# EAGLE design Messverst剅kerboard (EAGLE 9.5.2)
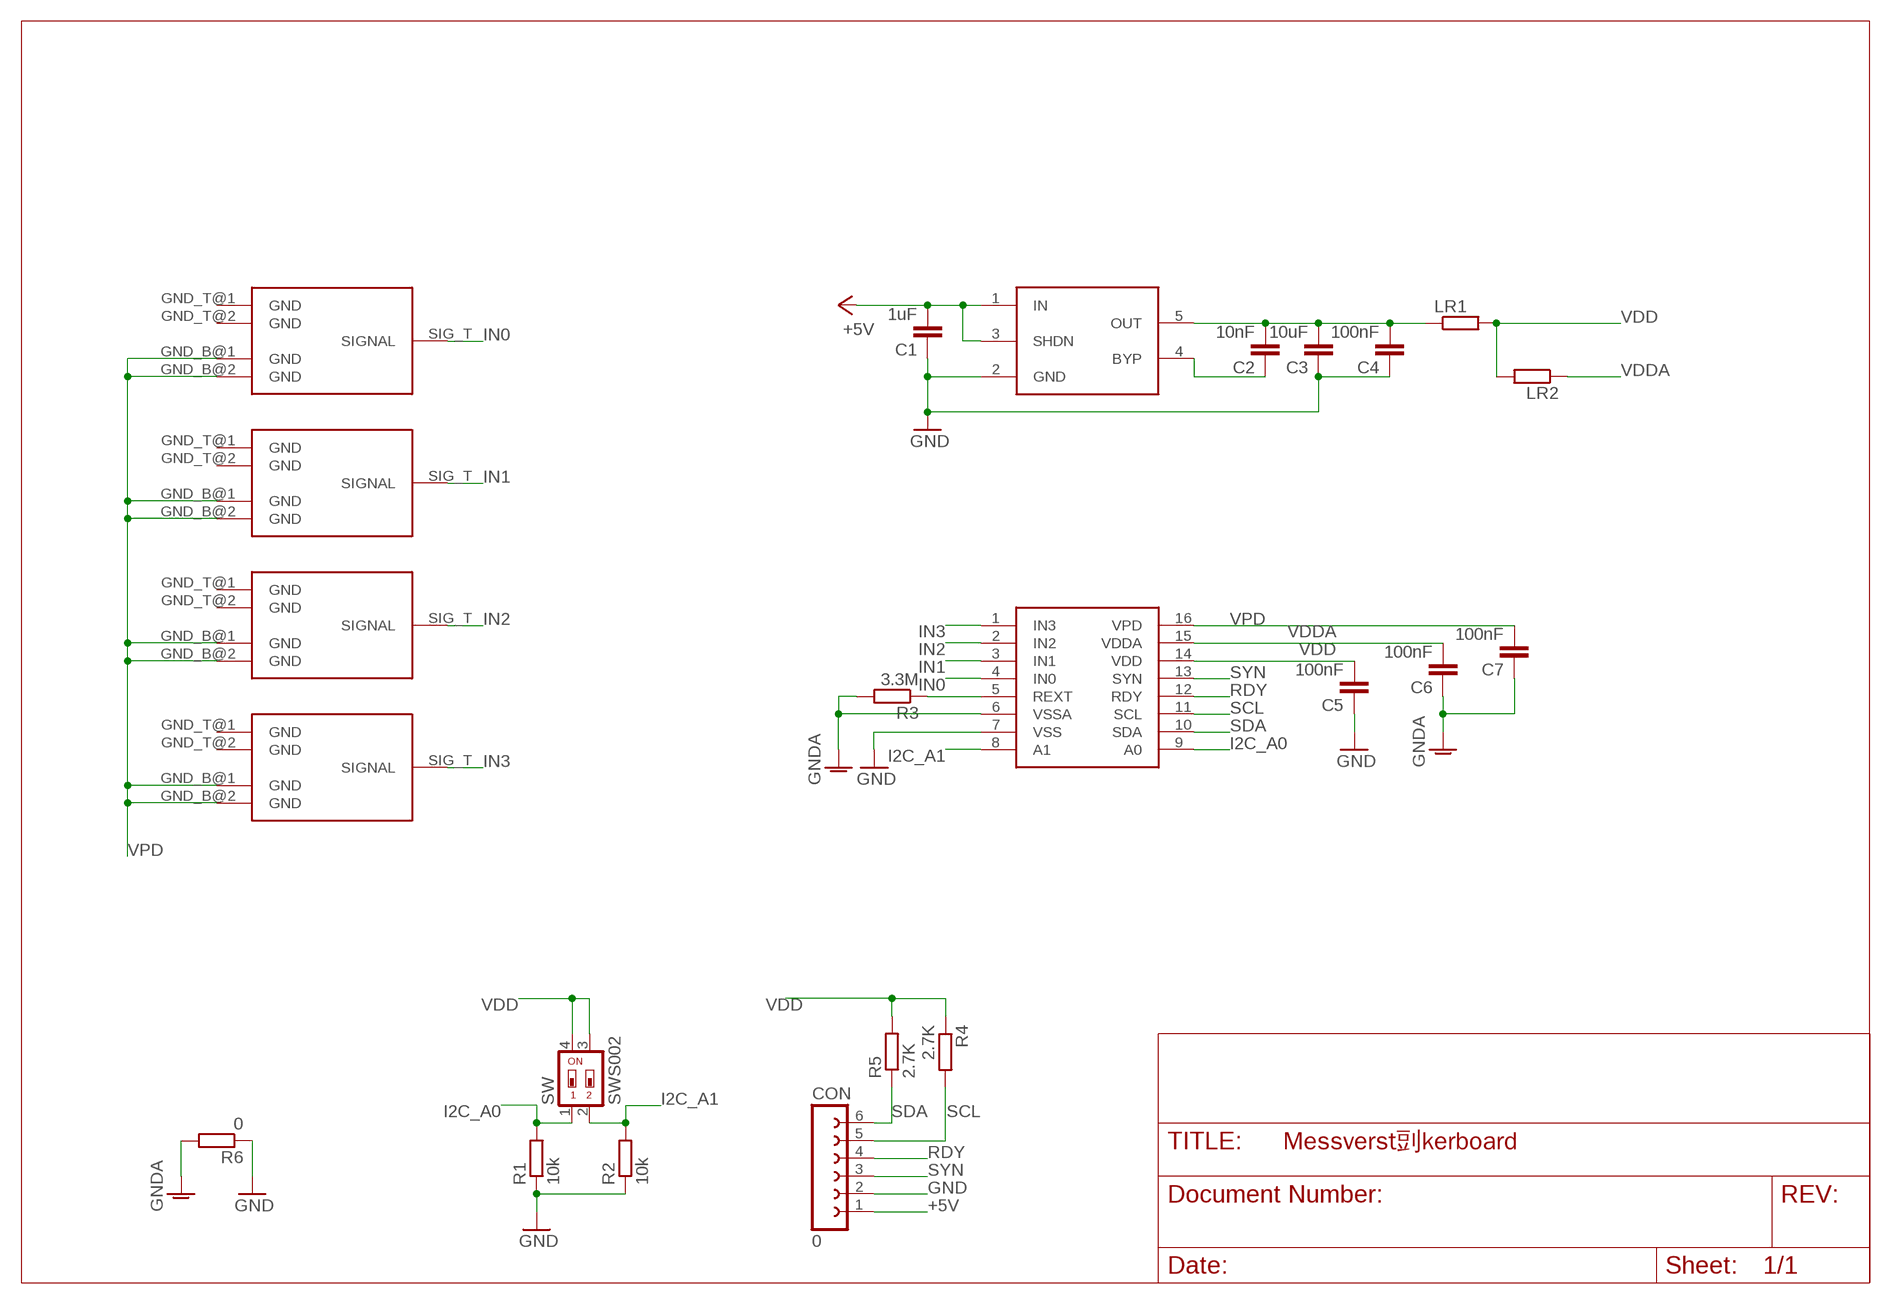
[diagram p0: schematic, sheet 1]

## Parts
AS89010  MCDC04  [SSOP16]
C1  1uF  C-EUC0603  [C0603]
C2  10nF  C-EUC0603  [C0603]
C3  10uF  C-EUC0603  [C0603]
C4  100nF  C-EUC0603  [C0603]
C5  100nF  C-EUC0603  [C0603]
C6  100nF  C-EUC0603  [C0603]
C7  100nF  C-EUC0603  [C0603]
CON  0  FE06-1  [FE06]
KANAL_1  SMA-BUCHSE-RANDMONTAGE  [SMA-RAND-PRINT]
KANAL_2  SMA-BUCHSE-RANDMONTAGE  [SMA-RAND-PRINT]
KANAL_3  SMA-BUCHSE-RANDMONTAGE  [SMA-RAND-PRINT]
KANAL_4  SMA-BUCHSE-RANDMONTAGE  [SMA-RAND-PRINT]
LDO  LT1761  [TSOT23-5]
LR1  R-EU_R0603  [R0603]
LR2  R-EU_R0603  [R0603]
R1  10k  R-EU_R0603  [R0603]
R2  10k  R-EU_R0603  [R0603]
R3  3.3M  R-EU_R0603  [R0603]
R4  2.7K  R-EU_R0603  [R0603]
R5  2.7K  R-EU_R0603  [R0603]
R6  0  R-EU_R0603  [R0603]
SW  SWS002  [SMS-002]

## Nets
+5V: C1.2 CON.1 LDO.1(IN) LDO.3(SHDN)
GND: AS89010.7(VSS) C1.1 C3.1 C4.1 C5.1 CON.2 LDO.2(GND) R1.1 R2.1 R6.1
GNDA: AS89010.6(VSSA) C6.1 C7.1 R3.2 R6.2
I2C_A0: AS89010.9(A0) R1.2 SW.1
I2C_A1: AS89010.8(A1) R2.2 SW.2
IN0: AS89010.4(IN0) KANAL_1.SIG_T(SIGNAL)
IN1: AS89010.3(IN1) KANAL_2.SIG_T(SIGNAL)
IN2: AS89010.2(IN2) KANAL_3.SIG_T(SIGNAL)
IN3: AS89010.1(IN3) KANAL_4.SIG_T(SIGNAL)
LDO_OUT3V3: C2.2 C3.2 C4.2 LDO.5(OUT) LR1.1
N$5: C2.1 LDO.4(BYP)
N$8: AS89010.5(REXT) R3.1
RDY: AS89010.12(RDY) CON.4
SCL: AS89010.11(SCL) CON.5 R4.2
SDA: AS89010.10(SDA) CON.6 R5.1
SYN: AS89010.13(SYN) CON.3
VDD: AS89010.14(VDD) C5.2 LR1.2 LR2.2 R4.1 R5.2 SW.3 SW.4
VDDA: AS89010.15(VDDA) C6.2 LR2.1
VPD: AS89010.16(VPD) C7.2 KANAL_1.GND_B@1(GND) KANAL_1.GND_B@2(GND) KANAL_2.GND_B@1(GND) KANAL_2.GND_B@2(GND) KANAL_3.GND_B@1(GND) KANAL_3.GND_B@2(GND) KANAL_4.GND_B@1(GND) KANAL_4.GND_B@2(GND)
Unconnected: KANAL_1.GND_T@1(GND) KANAL_1.GND_T@2(GND) KANAL_2.GND_T@1(GND) KANAL_2.GND_T@2(GND) KANAL_3.GND_T@1(GND) KANAL_3.GND_T@2(GND) KANAL_4.GND_T@1(GND) KANAL_4.GND_T@2(GND)

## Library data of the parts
AS89010 = BachelorLib:MCDC04
C1-C7 = rcl:C-EU: CAPACITOR, European symbol
CON = con-lsta:FE06-1: FEMALE HEADER; OC_FARNELL: unknown; OC_NEWARK: unknown
KANAL_1-KANAL_4 = OpenPhotonicsLib:SMA-BUCHSE-RANDMONTAGE
LDO = OpenPhotonicsLib:LT1761
LR1 LR2 R1-R6 = rcl:R-EU_: RESISTOR, European symbol
SW = smd-special:SWS002: SMD Dip Switch 2 pol.

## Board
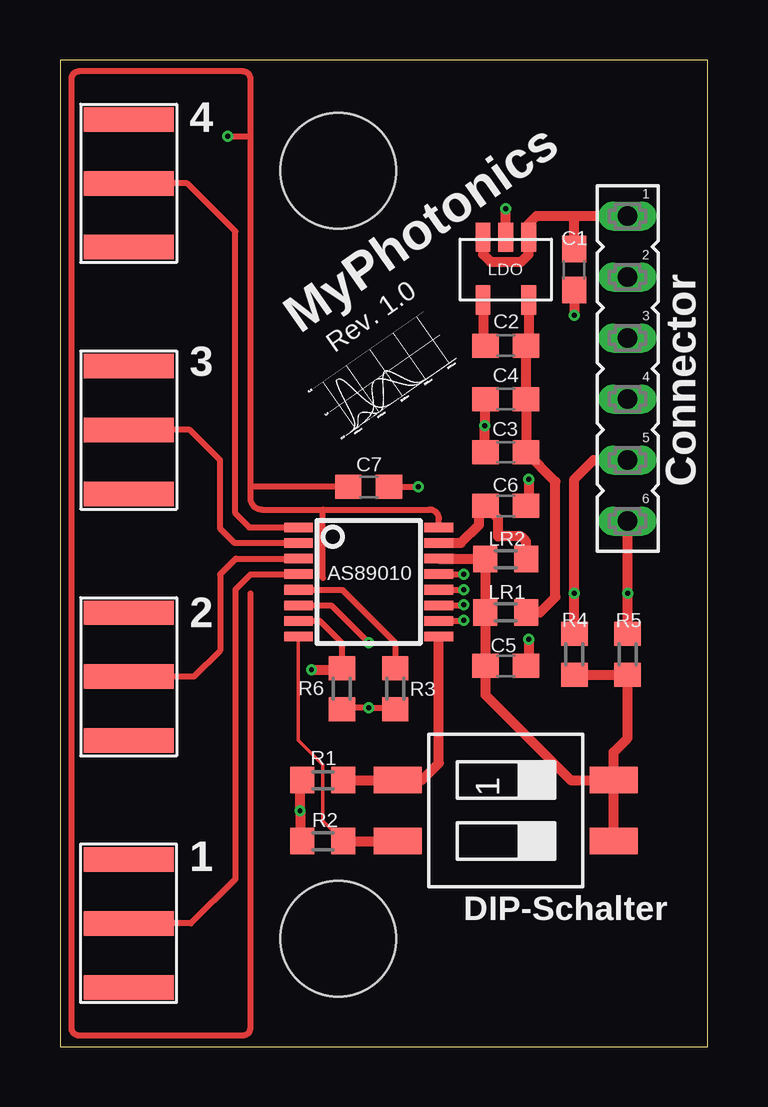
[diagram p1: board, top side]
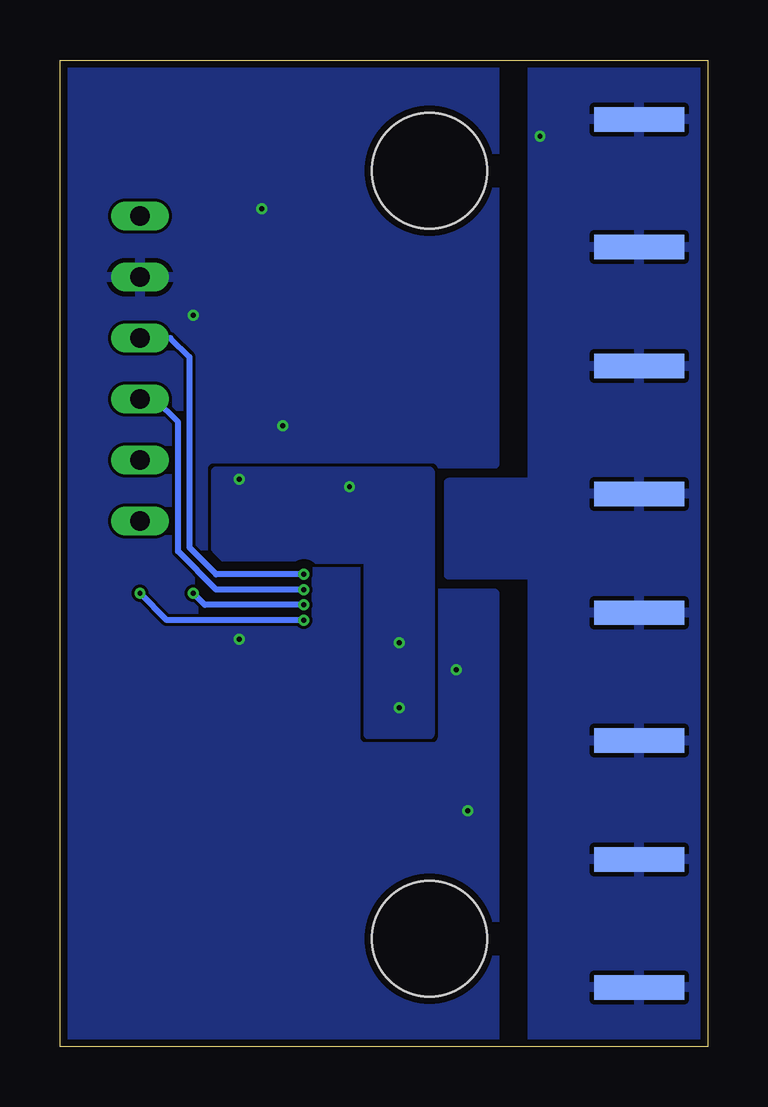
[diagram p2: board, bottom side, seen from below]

Size 26.99 x 41.12 mm. Coordinates in mm from the lower left corner, seen from the top.
Outline: 0,0 26.99,0 26.99,41.12 0,41.12 0,0
Copper layers (1+2*15+16): Top 0.035mm / dielectric 0.38mm / Route2 0.035mm / dielectric 0.71mm / Route15 0.035mm / dielectric 0.38mm / Bottom 0.035mm
Design rules "PCB-POOL HighSpec_ML4": minimum track width 0.125mm, minimum drill 0.2mm, track to track 0.125mm, track to pad 0.125mm, pad to pad 0.125mm, via to via 0.125mm, smd to smd 0.125mm, copper to edge 0.3mm, drill to drill 0.2mm, minimum pad ring 0.2mm, minimum via ring 0.125mm, stop-mask expansion 0.075mm, vias tented up to drill 0mil, thermal gap 0.2mm
Holes 4.8 mm at 11.6,36.5 11.6,4.5

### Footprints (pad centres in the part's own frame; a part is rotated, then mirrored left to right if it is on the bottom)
SSOP16 = smd 0.4 x 1.2: 1 -2.275,-2.925; 2 -1.625,-2.925; 3 -0.975,-2.925; 4 -0.325,-2.925; 5 0.325,-2.925; 6 0.975,-2.925; 7 1.625,-2.925; 8 2.275,-2.925; 9 2.275,2.925; 10 1.625,2.925; 11 0.975,2.925; 12 0.325,2.925; 13 -0.325,2.925; 14 -0.975,2.925; 15 -1.625,2.925; 16 -2.275,2.925
C0603 = smd 1.1 x 1: 1 -0.85,0; 2 0.85,0
FE06 = drill 0.813 long: 1 -6.35,0; 2 -3.81,0; 3 -1.27,0; 4 1.27,0; 5 3.81,0; 6 6.35,0
SMA-RAND-PRINT = smd 3.75 x 1.02 bottom: GND_B@1 0,2.665; GND_B@2 0,-2.665 | smd 3.75 x 1.02: GND_T@1 0,2.665; GND_T@2 0,-2.665; SIG_T 0,0
TSOT23-5 = smd 0.62 x 1.22: 1 0,-2.62; 2 0.95,-2.62; 3 1.9,-2.62; 4 1.9,0; 5 0,0
R0603 = smd 1 x 1.1: 1 -0.85,0; 2 0.85,0
SMS-002 = smd 1.092 x 2.007: 1 -1.27,-4.496; 2 1.27,-4.496; 3 1.27,4.496; 4 -1.27,4.496

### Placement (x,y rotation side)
AS89010  12.86,19.37 270 top
C1  21.43,32.38 90 top
C2  18.57,29.21 0 top
C3  18.57,24.77 0 top
C4  18.57,26.99 0 top
C5  18.57,15.88 180 top
C6  18.57,22.54 180 top
C7  12.86,23.34 180 top
CON  23.65,28.26 270 top
KANAL_1  2.86,5.14 180 top
KANAL_2  2.86,15.42 0 top
KANAL_3  2.86,25.7 0 top
KANAL_4  2.86,35.98 0 top
LDO  19.53,31.11 180 top
LR1  18.57,18.1 180 top
LR2  18.57,20.32 180 top
R1  10.95,11.11 0 top
R2  10.95,8.57 0 top
R3  13.97,14.92 270 top
R4  21.43,16.35 90 top
R5  23.65,16.35 270 top
R6  11.75,14.92 270 top
SW  18.57,9.84 270 top
U$1  [LOGO]  11.75,25.08 35 top

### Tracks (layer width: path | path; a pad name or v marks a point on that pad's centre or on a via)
+5V
  Top 0.406: 21.43,34.61 19.84,34.61 19.53,34.29 LDO.1 19.53,33.02 19.21,32.7 17.94,32.7 17.63,33.02 LDO.3 | C1.2 21.43,34.61 | CON.1 21.43,34.61
GND  (via drill 0.2 pad 0.25, 0.2 pad 0.41)
  Top 0.125: 10.32,8.57 R2.1 | 10.32,11.11 R1.1
  Top 0.152: 11.75,15.72 R6.1
  Top 0.254: AS89010.7 10.83,17.74 11.75,16.83 R6.1
  Top 0.406: R1.1 10,11.01 v10,9.84 10,8.68 R2.1 | v19.53,16.99 19.53,15.98 C5.1 | C3.1 17.7,24.79 v17.7,25.88 17.7,26.96 C4.1 | LDO.2 v18.57,34.92 | C1.1 v21.43,30.48 | v10.48,15.72 11.75,15.72
  pour Bottom (rank 2): 8.89,0 26.99,0 26.99,41.12 8.89,41.12 8.89,24.29 11.59,24.29 11.59,18.89 8.89,18.89
GNDA  (via drill 0.2 pad 0.25, 0.2 pad 0.41)
  Top 0.254: R6.2 11.8,14.13 v12.86,14.13 13.91,14.13 R3.2 | AS89010.6 11.29,18.39 v12.86,16.83 | C7.1 v14.92,23.34
  Top 0.406: v19.53,23.65 19.53,22.64 C6.1
  pour Bottom (isolate 0.406): 11.59,23.97 11.59,13.02 14.13,13.02 14.13,20.32 20.48,20.32 20.48,23.97
I2C_A0
  Top 0.406: R1.2 SW.1 15.08,11.11 15.78,11.81 AS89010.9
I2C_A1
  Top 0.152: R2.2 10.95,9.42 10.95,11.75 9.93,12.77 AS89010.8
  Top 0.406: R2.2 SW.2
IN0
  Top 0.254: AS89010.4 7.94,19.68 7.3,19.05 7.3,6.99 5.46,5.14 KANAL_1.SIG_T 2.91,5.08
IN1
  Top 0.254: AS89010.3 7.33,20.34 6.67,19.68 6.67,16.51 5.58,15.42 KANAL_2.SIG_T
IN2
  Top 0.254: AS89010.2 7.26,20.99 6.67,21.59 6.67,24.45 5.42,25.7 KANAL_3.SIG_T
IN3
  Top 0.254: AS89010.1 7.88,21.64 7.3,22.23 7.3,33.97 5.29,35.98 KANAL_4.SIG_T
LDO_OUT3V3
  Top 0.406: LDO.5 19.53,29.31 C2.2 C4.2 C3.2 20.64,23.55 20.64,18.73 20,18.1 LR1.1
N$5
  Top 0.406: LDO.4 17.63,29.31 C2.1
N$8
  Top 0.254: AS89010.5 11.76,19.04 13.97,16.83 R3.1
RDY  (via drill 0.2 pad 0.25)
  Top 0.254: AS89010.12 v16.82,19.04 arc90 v16.83,19.05
  Bottom 0.254: v16.83,19.05 20.48,19.05 22.07,20.64 22.07,26.04 23.02,26.99 CON.4
SCL  (via drill 0.2 pad 0.25)
  Top 0.254: AS89010.11 16.8,18.39 arc90 v16.83,18.41
  Top 0.406: R4.2 v21.43,18.89 21.43,23.65 22.23,24.45 CON.5
  Bottom 0.254: v16.83,18.41 20.95,18.41 v21.43,18.89
SDA  (via drill 0.2 pad 0.25)
  Top 0.254: AS89010.10 16.79,17.74 arc90 v16.83,17.78
  Top 0.406: R5.1 v23.65,18.89 CON.6
  Bottom 0.254: v16.83,17.78 22.54,17.78 v23.65,18.89
SYN  (via drill 0.2 pad 0.25)
  Top 0.254: AS89010.13 16.82,19.69 arc-90 v16.83,19.68
  Bottom 0.254: v16.83,19.68 20.48,19.68 21.59,20.8 21.59,28.73 22.38,29.53 CON.3
VDD
  Top 0.406: SW.3 SW.4 | R4.1 R5.2 23.65,12.86 23.07,12.28 SW.4 | AS89010.14 17.7,20.34 LR2.2 LR1.2 C5.2 17.72,14.66 21.27,11.11 SW.4
VDDA
  Top 0.406: AS89010.15 16.71,20.99 17.46,21.75 17.46,22.28 C6.2 | 17.62,22.44 C6.2 | LR2.1 19.42,21.06 19.21,21.27 18.26,21.27 18.26,22.01 C6.2
VPD  (via drill 0.2 pad 0.25)
  Top 0.254: AS89010.16 15.78,22 arc90 15.4,22.38 10.95,22.38 | 7.94,23.34 7.94,22.86 arc90 8.41,22.38 10.95,22.38 | 7.94,23.34 7.94,37.94 | 7.94,37.94 7.94,40.32 arc90 7.62,40.64 0.79,40.64 arc90 0.48,40.32 0.48,0.79 arc90 0.79,0.48 7.62,0.48 arc90 7.94,0.79 7.94,18.89 | C7.2 7.94,23.34 | v6.99,37.94 7.94,37.94 | 10.95,19.53 10.95,22.38
  pour Bottom (rank 3): 7.3,41.12 7.3,23.5 10.79,23.5 10.79,19.68 7.3,19.68 7.3,0 0,0 0,41.12

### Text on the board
tNames: 4 | LDO | MyPhotonics | Rev. 1.0 | 3 | Connector | 2 | 1 | DIP-Schalter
